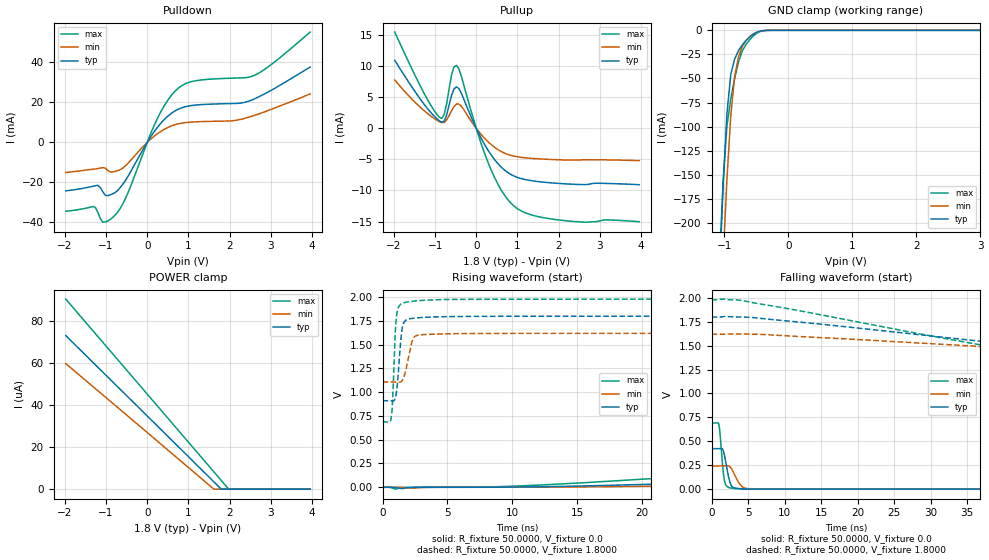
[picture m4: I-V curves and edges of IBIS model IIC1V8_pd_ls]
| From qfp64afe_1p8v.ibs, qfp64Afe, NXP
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[Model] IIC1V8_pd_ls
|   Model IIC1V8_pd_ls
| This model was characterised for following simulation conditions:
| External (pad) voltage:
|   - Typ: 1.8V,   - Min: 1.62V,   - Max: 1.98V
| Library cells for typ/min/max conditions are connected as defined below:
|  IO - External Pad
|  A - Core Input
|  EN - Output Buffer Enable
|  BOOST - vdde
|  EGP - vdd
|  EHS - gnd
|  ENZI - vdd
|  EPD - vdd
|  EPUN - vdd
|  ZI - NC
|  ZIF - NC
|  gnd - gnd
|  gnde - gnde
|  vdd - vdd
|  vdde - vdde
| All other pins connected to ground
Model_type I/O
Polarity   Non-Inverting
Enable   Active-Low
Vinl =   0.5400V
Vinh =   1.2600V
Vmeas =  0.9000V
Cref =   0.0F
Rref =   1.0000k
Vref =   0.0V
C_comp   3.6136pF   3.4665pF   3.7543pF
|C_comp_pullup   0.9376pF   0.9156pF   0.9440pF
|C_comp_pulldown   2.3254pF   2.4783pF   2.1797pF
[Model Spec]
| variable   typ   min   max
Vinh   0.5400V   0.4860V   0.5940V
Vinl   1.2600V   1.1340V   1.3860V
Vmeas   0.9000V   0.8100V   0.9900V
[Temperature Range]   25.0000   0.1250k   -40.0000
[Voltage Range]   1.8000V   1.6200V   1.9800V
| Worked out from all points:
|   slope of the pulldown table from 0 to 0.27 V, typ, clamps not added: 33.4 ohm
|   slope of the pullup table from 0 to 0.27 V, typ, clamps not added: 80.7 ohm
|   GND clamp passes 1 mA (typ) near -0.44 V on its own axis
|   rising waveform, R_fixture 50.0000, V_fixture 0.0: 20-80 % time 70.1ns typ, 81.9ns min, 57ns max; typ from 0 V to 0.423 V
|   rising waveform, R_fixture 50.0000, V_fixture 1.8000: 20-80 % time 318ps typ, 487ps min, 235ps max; typ from 0.91 V to 1.8 V
|   falling waveform, R_fixture 50.0000, V_fixture 0.0: 20-80 % time 671ps typ, 1.04ns min, 474ps max; typ from 0.423 V to 0 V
|   falling waveform, R_fixture 50.0000, V_fixture 1.8000: 20-80 % time 66.9ns typ, 88.6ns min, 48.9ns max; typ from 1.8 V to 0.91 V
[Pulldown]
|Voltage   I(typ)   I(min)   I(max)
-1.98V    -24.22mA   -15.04mA   -34.42mA
-1.32V    -21.94mA   -13.4mA    -32.06mA
-1.2V     -21.45mA   -13.05mA   -35.06mA
-1.08V    -24.63mA   -12.6mA    -39.9mA
-900mV    -26.23mA   -14.78mA   -38.53mA
-720mV    -24.07mA   -14.13mA   -34.99mA
-540mV    -19.33mA   -11.9mA    -28.53mA
300mV     8.856mA    5.096mA    14.12mA
720mV     16.26mA    9.117mA    26.48mA
1.14V     18.6mA     10.26mA    30.69mA
2.58V     21.55mA    13.34mA    33.32mA
3.96V     37.7mA     24.26mA    55.17mA
[Pullup]
|Voltage   I(typ)   I(min)   I(max)
-1.98V    10.93mA    7.779mA    15.48mA
-1.32V    4.332mA    3.147mA    6.287mA
-900mV    1.21mA     1.087mA    1.795mA
-780mV    1.15mA     923.8uA    2.217mA
-600mV    5.282mA    2.828mA    8.607mA
-480mV    6.665mA    3.904mA    10.12mA
-420mV    6.371mA    3.888mA    9.538mA
360mV     -4.265mA   -2.608mA   -6.666mA
660mV     -6.57mA    -3.917mA   -10.5mA
960mV     -7.8mA     -4.537mA   -12.74mA
2.04V     -8.889mA   -5.075mA   -14.77mA
3.96V     -9.081mA   -5.209mA   -15.04mA
[GND_clamp]
|Voltage   I(typ)   I(min)   I(max)
-1.98V    -2.104A    -2.075A    -2.136A
-1.08V    -259.3mA   -333mA     -246.9mA
-1.02V    -161.8mA   -238.7mA   -157.1mA
-960mV    -86.75mA   -154.7mA   -99.47mA
-900mV    -45.96mA   -88.82mA   -71.06mA
-840mV    -29.91mA   -48mA      -50.26mA
-780mV    -21.16mA   -27.65mA   -32.99mA
-720mV    -15.17mA   -16.88mA   -21.27mA
-660mV    -10.57mA   -10.24mA   -14.57mA
-540mV    -3.796mA   -3.405mA   -5.301mA
-300mV    -21.69uA   -40.85uA   -23.15uA
3.96V     0A         0A         0A
[POWER_clamp]
|Voltage   I(typ)   I(min)   I(max)
-1.98V    73.06uA    59.72uA    90.42uA
1.62V     3.484uA    0A         8.225uA
1.8V      0A         0A         4.113uA
1.98V     0A         0A         0A
3.96V     0A         0A         0A
[Ramp]
| variable   typ   min   max
dV/dt_r  0.2537/70.0854n   0.1455/81.9074n   0.4146/57.0196n
dV/dt_f  0.5332/66.9137n   0.3065/88.6388n   0.7749/48.9047n
R_load = 50.0000
[Rising Waveform]
R_fixture= 50.0000
V_fixture= 0.0
V_fixture_min= 0.0
V_fixture_max= 0.0
|time   V(typ)   V(min)   V(max)
0s        583.8pV    50.78nV    39.11pV
1.014ns   -3.352mV   193.4uV    -19.98mV
1.639ns   -11.12mV   -2.819mV   -1.762mV
12.78ns   6.528mV    1.462mV    27.86mV
46.58ns   148.4mV    66.48mV    309.9mV
85.13ns   286.8mV    144.3mV    563.6mV
105.2ns   344.5mV    174.6mV    633mV
135.4ns   393.2mV    208.9mV    672.9mV
252ns     422mV      241.1mV    690.6mV
1us       422.8mV    242.6mV    690.9mV
[Rising Waveform]
R_fixture= 50.0000
V_fixture= 1.8000
V_fixture_min= 1.6200
V_fixture_max= 1.9800
|time   V(typ)   V(min)   V(max)
0s        910.3mV    1.108V     687.5mV
676.2ps   909mV      1.108V     736.1mV
774.3ps   906.6mV    1.108V     908.1mV
1.008ns   951.3mV    1.107V     1.695V
1.272ns   1.31V      1.104V     1.904V
1.481ns   1.641V     1.117V     1.931V
1.772ns   1.754V     1.219V     1.944V
2.539ns   1.78V      1.59V      1.96V
5.798ns   1.796V     1.615V     1.976V
1us       1.799V     1.619V     1.979V
[Falling Waveform]
R_fixture= 50.0000
V_fixture= 0.0
V_fixture_min= 0.0
V_fixture_max= 0.0
|time   V(typ)   V(min)   V(max)
0s        422.9mV    242.6mV    691mV
1.007ns   422.8mV    242.6mV    674.8mV
1.156ns   424.2mV    242.6mV    584.4mV
1.623ns   397.6mV    242.6mV    164mV
1.945ns   278.8mV    244.2mV    43.83mV
2.356ns   118.8mV    241.4mV    17.71mV
2.769ns   31.22mV    208.6mV    9.848mV
4.018ns   4.358mV    38.89mV    3.101mV
5.084ns   1.766mV    4.84mV     1.766mV
1us       18.99nV    83.33nV    10.91nV
[Falling Waveform]
R_fixture= 50.0000
V_fixture= 1.8000
V_fixture_min= 1.6200
V_fixture_max= 1.9800
|time   V(typ)   V(min)   V(max)
0s        1.799V     1.619V     1.979V
4.118ns   1.799V     1.622V     1.972V
58.01ns   1.392V     1.406V     1.243V
67.61ns   1.331V     1.372V     1.005V
75.57ns   1.278V     1.346V     874.6mV
89.55ns   1.134V     1.304V     769.4mV
112.5ns   988mV      1.233V     712.2mV
147.5ns   929mV      1.144V     692.3mV
206.5ns   912.9mV    1.113V     688mV
1us       910.4mV    1.108V     687.5mV
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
